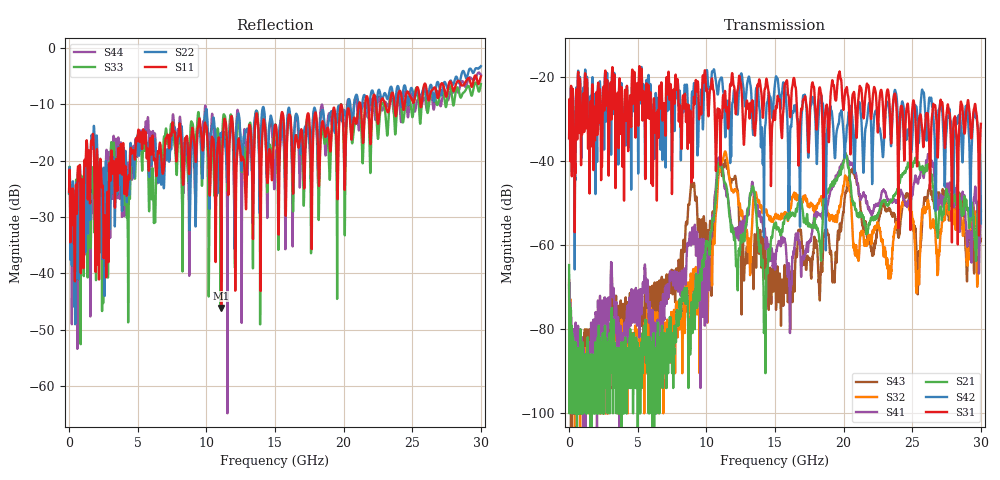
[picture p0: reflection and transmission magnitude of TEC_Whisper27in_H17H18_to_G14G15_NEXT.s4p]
! Tyco Electronics
! H17H18-G14G15_NEXT
!! PART DESCRIPTION: Whisper 27in Megtron 6 VLP-HVLP-VLP Channel Model, bulkhead 2.4mm test pts
!! MODEL DESCRIPTION: System 4-port S-parameter
!! MODEL STATUS: Measured
!! MODEL GEOMETRY: Channel Model
!! MODEL FREQUENCY RANGE: DC to 30.000 GHz in 10.000 MHz frequency steps
!! MODEL EDGE RATE LIMITATION: 12.500 ps (Using conservative 0.5/Fmax rule of thumb)
!! TIME-DOMAIN TRANSFORM CAUTIONS:
!! 1.) Do not simulate transient edge rates faster than the number listed above.  Edge rates faster than this number
!!  contain significant spectral content at frequencies above the model's highest frequency.
!! 2.) Even when simulating edge rates that are slower than the number listed above, be aware that the best time
!!  resolution possible with a direct iFFT is (1 / 2Fmax).  As a result, time resolution is typically not adequate
!!  for most time-domain simulations unless tricks such as windowing are used to minimize leakage and aliasing.
!! 3.) Because the model has a uniform frequency step, a direct iFFT will result in an impulse that that has a time
!!  length given by either (1 / Fstep) or (1 / 2Fstep), depending on the transform being used.  Care has been taken
!!  in selecting the frequency step to ensure a settled impulse response for the model.  Therefore, convolution with
!!  the model's impulse response should present no issues.  However, if directly concatenating s-parameter models
!!  in the frequency domain a user must either interpolate necessary interim frequencies or complete impulse response
!!  zero-padding.  Impulse response zero-padding is more difficult, but more accurate.
!! PORT DEFINITIONS:
!! Port  1  ----->  Side A  H17  G14  Side A  <-----  Port  2
!! Port  3  ----->  Side A  H18  G15  Side A  <-----  Port  4
! Point-to-Point link (differential)  !
! Connectors:  !
!  1: STRADA Whisper  !
! Materials:  !
!  Backplane: Megtron-6 HVLP  !
!  Daughtercard: Megtron-6 VLP  !
! Stack-up:  !
!  Backplane: 20 layers, 200mil thick  !
!  Daughtercard: 14 layers, 110mil thick  !
! Trace Length:  !
!  Backplane: 17in  !
!  Daightercards: 5in  !
! Trace Width:  !
!  Backplane: 8-13-8 mils  !
!  Daughtercards: 6-9-6 mils  !
! Geometry:  !
!  Backplane: Stripline  !
!  Daughtercards: Stripline  !
! Freq. Range: 0 GHz - 30 GHz  !
! Note1: non-mixed-mode s-parameters  !
! Note2: channel includes 2.4mm test points  !
! Touchstone data converted from IdEM dataset
# GHz S MA R 50
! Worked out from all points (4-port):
!   3000 points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, 10 MHz to 30 GHz, reference 50 ohm
!   strongest paths, dB at 10 MHz, 7.51 GHz, 15.01 GHz, 22.51 GHz, 30 GHz:
!     S31: -34.6, -43.9, -30.1, -32.8, -31.1
!     S42: -34.5, -34.3, -21.3, -30.6, -54.8
!     S21: -64.7, -90.5, -55.7, -52.7, -51.9
!     S41: -69.6, -66.4, -65.8, -50.3, -51.8
!     S32: -68.2, -77.7, -53.2, -55.2, -54.0
!     S43: -69.1, -68.9, -65.2, -55.1, -58.5
!   lowest |S11| = -46.2 dB at 11.09 GHz (marker M1), VSWR 1.01, Z = 49.5 - j0.0541 ohm
!   |S11| at or under -10 dB: start of sweep to 21.11 GHz; 21.23 GHz to 21.58 GHz (349.3 MHz wide, 1.63 % of centre); 23.02 GHz to 23.37 GHz (347.4 MHz wide, 1.5 % of centre)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
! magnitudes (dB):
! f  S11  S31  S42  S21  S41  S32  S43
! 10 MHz  -25.5  -34.6  -34.5  -64.7  -69.6  -68.2  -69.1
! 5.35 GHz  -17.0  -29.4  -27.4  -88.0  -70.8  -86.0  -74.9
! 8.81 GHz  -19.2  -31.9  -33.2  -80.0  -57.1  -73.2  -48.5
! 11.09 GHz  -46.2  -30.0  -20.1  -41.2  -40.7  -40.6  -41.1
! 14.3 GHz  -14.8  -22.6  -31.5  -84.4  -58.6  -51.9  -60.2
! 20.12 GHz  -21.5  -23.3  -36.5  -38.5  -38.3  -43.4  -47.9
! 30 GHz  -5.1  -31.1  -54.8  -51.9  -51.8  -54.0  -58.5
